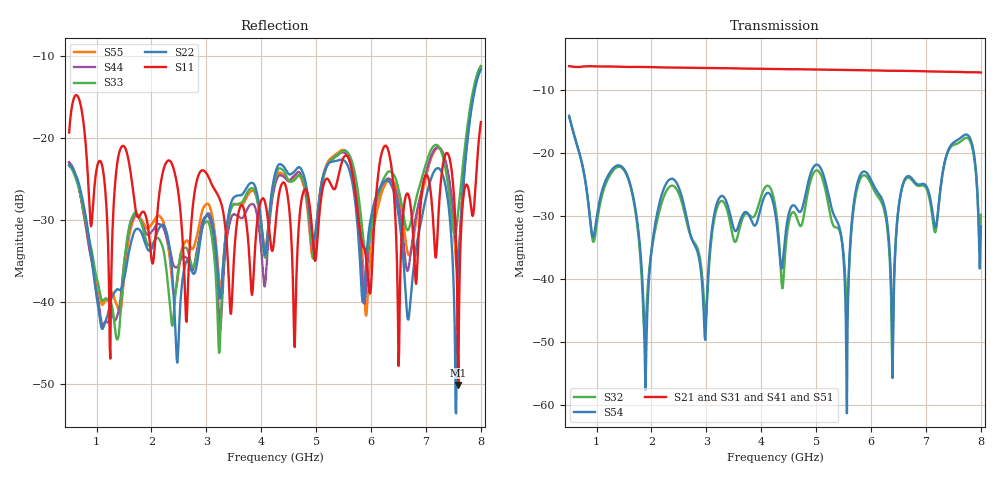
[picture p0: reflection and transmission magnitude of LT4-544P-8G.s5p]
! MTS Systemtechnik GmbH
! S-Parameters
! Model: LT4-544P-8G
! Rohde & Schwarz ZVB8 2Ports - Version 3.20 - 1145.1010k08 SN: 100119
! Converted & adapted with Octave
!		|  MTS  |
!		|  |--o OUT 4 (Port 5)
!		|  |--o OUT 3 (Port 4)
! C (Port 1) o--| LT4-544P-8G |
!  |  |--o OUT 2 (Port 3)
!  |  |--o OUT 1 (Port 2)
! S5P File: Measurements:
! <S11,S12,S13,S14,S15>,
! <S21,S22,S23,S24,S25>,
! <S31,S32,S33,S34,S35>,
! <S41,S42,S43,S44,S45>,
! <S51,S52,S53,S54,S55>:
# HZ  S  DB  R  50.00
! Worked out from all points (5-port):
!   751 points, 500 MHz to 8 GHz, reference 50 ohm
!   strongest paths, dB at 500 MHz, 2.37 GHz, 4.25 GHz, 6.13 GHz, 8 GHz:
!     S21: -6.3, -6.5, -6.7, -6.9, -7.3
!     S31: -6.3, -6.5, -6.7, -7.0, -7.4
!     S41: -6.2, -6.5, -6.7, -7.0, -7.3
!     S51: -6.2, -6.5, -6.8, -7.0, -7.4
!     S54: -14.2, -24.1, -29.3, -26.3, -31.6
!     S32: -14.1, -25.2, -28.2, -27.0, -29.8
!   lowest |S11| = -50.1 dB at 7.59 GHz (marker M1), VSWR 1.01, Z = 49.8 + j0.247 ohm
!   |S11| at or under -10 dB: start of sweep to end of sweep
